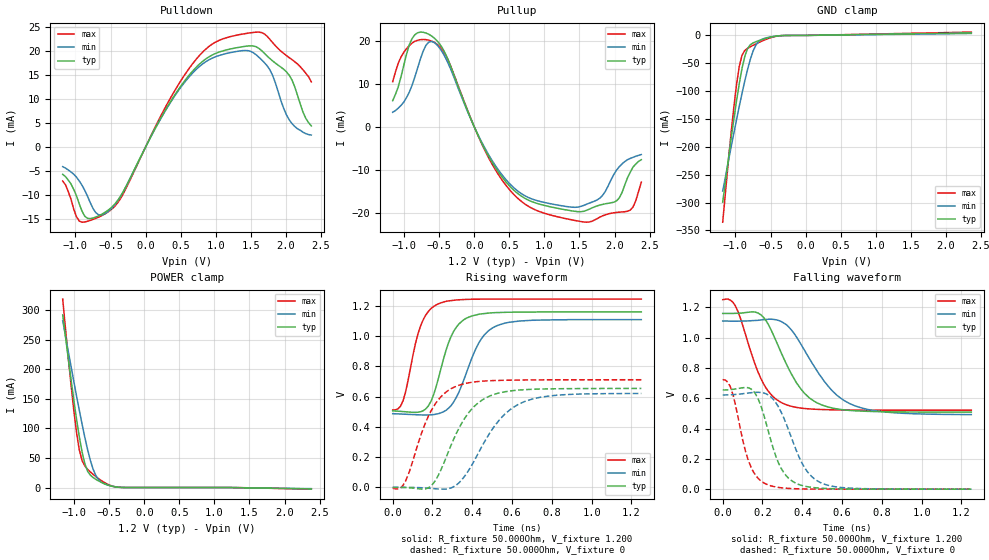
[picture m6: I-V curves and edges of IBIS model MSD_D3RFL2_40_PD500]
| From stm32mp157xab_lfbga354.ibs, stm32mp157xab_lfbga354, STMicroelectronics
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[Model] MSD_D3RFL2_40_PD500
Model_type   I/O
C_comp 2.418pF   2.333pF   2.542pF
Vinh = 820.000mV
Vinl = 380.000mV
Vmeas = 600.000mV
Vref = 600.000mV
[Model Spec]
Vinh   820.000mV   790.000mV   870.000mV
Vinl   380.000mV   350.000mV   430.000mV
Vmeas   600.000mV   570.000mV   650.000mV
Vref   600.000mV   570.000mV   650.000mV
[Temperature Range]   25.000   125.000   -40.000
[Voltage Range]   1.200V   1.140V   1.300V
[GND Clamp Reference]   0.00V   0.00V   0.00V
[Pulldown Reference]   0.00V   0.00V   0.00V
[POWER Clamp Reference]   1.200V   1.140V   1.300V
[Pullup Reference]   1.200V   1.140V   1.300V
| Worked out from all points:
|   slope of the pulldown table from 0 to 0.18 V, typ, clamps not added: 35.6 ohm
|   slope of the pullup table from 0 to 0.18 V, typ, clamps not added: 29.6 ohm
|   GND clamp passes 1 mA (typ) near -0.40 V on its own axis
|   POWER clamp passes 1 mA (typ) near -0.41 V on its own axis
|   rising waveform, R_fixture 50.000Ohm, V_fixture 1.200: 20-80 % time 94.2ps typ, 121ps min, 80.9ps max; typ from 0.506 V to 1.16 V
|   rising waveform, R_fixture 50.000Ohm, V_fixture 0: 20-80 % time 154ps typ, 187ps min, 131ps max; typ from 0.001 V to 0.655 V
|   falling waveform, R_fixture 50.000Ohm, V_fixture 1.200: 20-80 % time 157ps typ, 198ps min, 124ps max; typ from 1.16 V to 0.508 V
|   falling waveform, R_fixture 50.000Ohm, V_fixture 0: 20-80 % time 98.4ps typ, 123ps min, 82.6ps max; typ from 0.654 V to 0 V
[GND Clamp]
-1.182V   -299.2mA   -279.4mA   -335.3mA
-1.064V   -187.1mA   -201.6mA   -177.2mA
-984.9mV  -117.6mA   -151.5mA   -88.27mA
-945.5mV  -86.31mA   -127.1mA   -55.47mA
-906.1mV  -58.92mA   -103.8mA   -35.36mA
-866.7mV  -37.41mA   -81.56mA   -26.95mA
-787.9mV  -16.78mA   -42.84mA   -20.37mA
-709.1mV  -11.29mA   -17.41mA   -15.26mA
-630.3mV  -7.777mA   -7.464mA   -10.57mA
-512.1mV  -3.515mA   -2.998mA   -4.657mA
-315.1mV  -159.9uA   -226.2uA   -149.3uA
2.364V    4.576mA    3.518mA    5.996mA
[Power Clamp]
-1.164V   292.1mA    282.3mA    318.9mA
-1.085V   218.4mA    230.6mA    219.7mA
-1.006V   148.2mA    179.8mA    130.8mA
-966.7mV  115.7mA    154.9mA    93.06mA
-927.3mV  85.9mA     130.7mA    63.72mA
-887.9mV  60.18mA    107.2mA    45.62mA
-809.1mV  27.64mA    64.14mA    30.93mA
-730.3mV  16.89mA    31.01mA    22.25mA
-690.9mV  13.81mA    20.19mA    18.4mA
-572.7mV  6.565mA    6.472mA    8.682mA
-336.4mV  180.4uA    344.1uA    207.9uA
2.382V    -2.355mA   -1.942mA   -2.793mA
[Pulldown]
-1.182V   -5.7mA     -4.1mA     -7.1mA
-945.5mV  -11.91mA   -7.1mA     -15.47mA
-866.7mV  -14.47mA   -9.06mA    -15.66mA
-709.1mV  -14.63mA   -13.73mA   -14.9mA
-551.5mV  -13.37mA   -13.65mA   -13.72mA
-354.6mV  -10.22mA   -10.29mA   -10.71mA
590.9mV   14.46mA    14.13mA    15.79mA
945.5mV   19.18mA    18.52mA    21.45mA
1.339V    20.84mA    20.05mA    23.47mA
1.733V    19.01mA    16.98mA    23.14mA
2.009V    15.7mA     6.74mA     19.1mA
2.364V    4.4mA      2.5mA      13.6mA
[Pullup]
-1.164V   6.1mA      3.409mA    10.51mA
-887.9mV  20.5mA     9.662mA    19.46mA
-730.3mV  21.97mA    17.56mA    20.29mA
-612.1mV  21.14mA    19.84mA    19.93mA
-375.8mV  15.67mA    14.87mA    15.59mA
215.2mV   -7.105mA   -6.742mA   -7.481mA
727.3mV   -16.61mA   -16.01mA   -17.94mA
1.515V    -19.66mA   -18.45mA   -21.93mA
1.791V    -18.11mA   -16.51mA   -20.92mA
1.988V    -17.46mA   -11.08mA   -19.92mA
2.224V    -10.5mA    -7.295mA   -19.28mA
2.382V    -7.6mA     -6.395mA   -12.82mA
[Ramp]
R_load=50.000Ohm
dV/dt_r   392.070mV/124.500ps  372.209mV/155.000ps  431.040mV/106.000ps
dV/dt_f   392.070mV/128.500ps  372.179mV/162.500ps  431.040mV/103.500ps
[Rising waveform]
R_fixture=50.000Ohm
V_fixture=1.200
V_fixture_min=1.140
V_fixture_max=1.300
0s        505.9mV    487.7mV    512mV
52ps      501.7mV    484.8mV    573.1mV
115ps     496.3mV    480.9mV    954.6mV
154ps     507.7mV    479.2mV    1.11V
230ps     722.1mV    487.8mV    1.214V
281ps     957.6mV    524.4mV    1.233V
332ps     1.079V     627.2mV    1.24V
435ps     1.145V     959.6mV    1.244V
524ps     1.156V     1.069V     1.245V
1.25ns    1.16V      1.109V     1.245V
[Rising waveform]
R_fixture=50.000Ohm
V_fixture=0
0s        823.6uV    784.3uV    -5.389mV
64ps      -78.4uV    806uV      41.17mV
192ps     9.531mV    -6.01mV    504.3mV
320ps     357.6mV    16.54mV    669.2mV
383ps     496.3mV    115.7mV    692mV
447ps     575.3mV    267.9mV    702.2mV
537ps     624.9mV    447.7mV    707.7mV
639ps     644.3mV    553.8mV    710mV
817ps     652.3mV    608.7mV    711.5mV
1.25ns    654.6mV    621.2mV    711.9mV
[Falling waveform]
R_fixture=50.000Ohm
V_fixture=1.200
V_fixture_min=1.140
V_fixture_max=1.300
0s        1.159V     1.109V     1.25V
64ps      1.16V      1.108V     1.208V
192ps     1.15V      1.116V     729.6mV
243ps     1.051V     1.121V     624.2mV
307ps     862.3mV    1.096V     563.7mV
435ps     602.6mV    863.5mV    529.5mV
537ps     539.7mV    669.1mV    523.9mV
639ps     519.3mV    564.2mV    521.7mV
817ps     510.7mV    508.9mV    520.6mV
1.25ns    507.8mV    491.9mV    520.5mV
[Falling waveform]
R_fixture=50.000Ohm
V_fixture=0
0s        654.1mV    621.2mV    722.5mV
52ps      658.8mV    623.6mV    622.2mV
141ps     662.3mV    636mV      149.1mV
179ps     592.6mV    639mV      69.86mV
218ps     436.9mV    629mV      33.72mV
269ps     210mV      567mV      13.96mV
320ps     87.59mV    428.9mV    6.034mV
409ps     20.81mV    147.4mV    1.413mV
498ps     6.022mV    39.35mV    353.8uV
1.25ns    2.658uV    24.36uV    811.3nV
